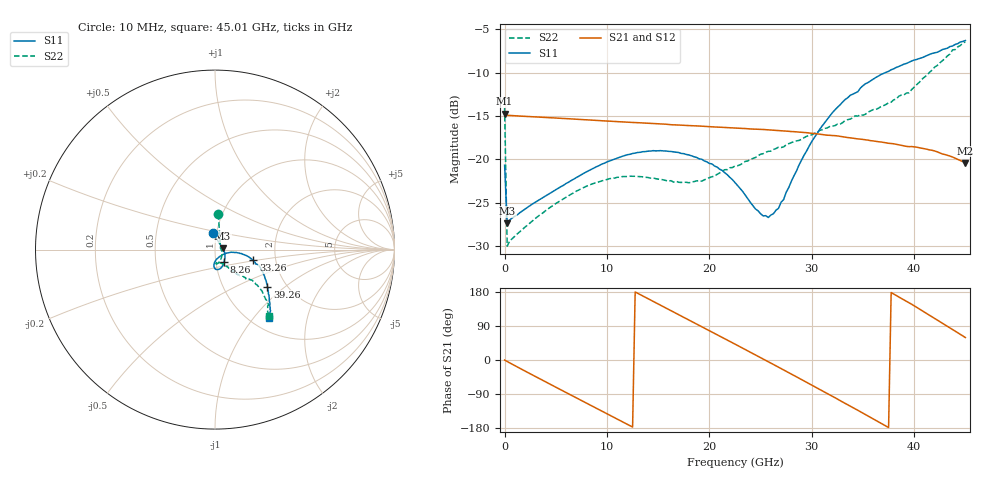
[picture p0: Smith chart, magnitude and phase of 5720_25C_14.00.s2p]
! Device:  ADRF5720
! Description: 0.5dB LSB GaAs MMIC 6-bit Digital Attenuator
! Frequency:  0.000009 -  40 GHz
! Ports:
!	RF1	= Port 1
!	RF2	= Port 2
! Vdd:  3.3 Volt
! Vss:  -3.3 Volt
! Control:  0/3.3 Volt
! State:  14.00 dB attenuation
! Data:  The device was measured using G-S-G Probes on a matrix board.
!  Data was collected using an calibrated 4 port network analyzer.
!  The reference plane for this measurement is at the launchers.
! Note:  Analog Devices supplies this data as a sample of measured data
!  for this product.  Your particular data for this product may vary.
!  Data was taken at 25 degrees C.
!  Analog Devices reserves the right to change this data at anytime.
# GHZ S DB R 45.0
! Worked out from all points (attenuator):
!   181 points, 10 MHz to 45.01 GHz, reference 45 ohm
!   highest |S21| = -14.71 dB at 10 MHz (marker M1); lowest = -20.4 dB at 45.01 GHz (marker M2)
!   lowest |S11| = -27.4 dB at 260 MHz (marker M3), VSWR 1.09, Z = 49 + j0.802 ohm
!   |S11| at or under -10 dB: start of sweep to 37.15 GHz
!   |S22| runs from -30.0 to -6.4 dB; largest |S21 - S12| = 0.00022
!   S11 on the Smith chart (normalised r, x): 10 MHz: 0.96, +0.18; 8.26 GHz: 1.10, -0.15; 33.26 GHz: 1.53, -0.19; 39.26 GHz: 1.60, -0.76; 45.01 GHz: 1.21, -1.21
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0.01  -20.66 96.5  -14.71 -0.1  -14.71 -0.1  -14.04 84.6
0.26  -27.35 11.0  -14.90 -4.0  -14.91 -4.0  -30.00 13.9
1.26  -26.37 -3.0  -14.97 -18.5  -14.98 -18.5  -28.57 -7.4
4.26  -24.02 -29.0  -15.17 -61.1  -15.17 -61.1  -25.70 -42.8
7.76  -21.58 -50.6  -15.41 -110.4  -15.41 -110.4  -23.22 -66.3
8.26  -21.27 -53.2  -15.44 -117.4  -15.44 -117.4  -22.97 -68.5
11.76  -19.54 -69.6  -15.68 -166.5  -15.69 -166.4  -21.97 -81.2
15.26  -18.98 -82.6  -15.90 144.3  -15.90 144.3  -22.30 -84.7
19.01  -19.93 -92.0  -16.14 91.5  -16.15 91.5  -22.45 -72.1
21.26  -21.26 -93.8  -16.29 59.6  -16.29 59.6  -21.34 -64.3
22.76  -23.00 -92.0  -16.39 38.4  -16.39 38.4  -20.72 -60.1
24.51  -25.71 -75.6  -16.50 13.5  -16.50 13.6  -19.77 -57.3
25.76  -26.69 -52.4  -16.58 -4.5  -16.58 -4.5  -19.06 -55.9
27.26  -24.62 -22.2  -16.70 -26.3  -16.70 -26.2  -18.55 -53.4
28.76  -20.64 -9.2  -16.84 -48.0  -16.84 -47.9  -17.80 -52.6
30.26  -17.47 -7.9  -17.01 -70.0  -17.02 -70.0  -16.98 -51.0
33.26  -13.09 -15.7  -17.43 -114.3  -17.43 -114.3  -15.51 -48.5
35.51  -11.12 -23.1  -17.77 -148.0  -17.77 -147.9  -14.53 -47.1
37.76  -9.65 -30.9  -18.16 178.1  -18.16 178.1  -13.39 -43.4
39.26  -8.92 -35.4  -18.49 154.8  -18.49 154.9  -12.33 -42.5
42.26  -7.63 -43.3  -19.12 105.5  -19.12 105.5  -9.16 -41.4
45.01  -6.27 -51.5  -20.39 59.3  -20.38 59.3  -6.41 -50.9
